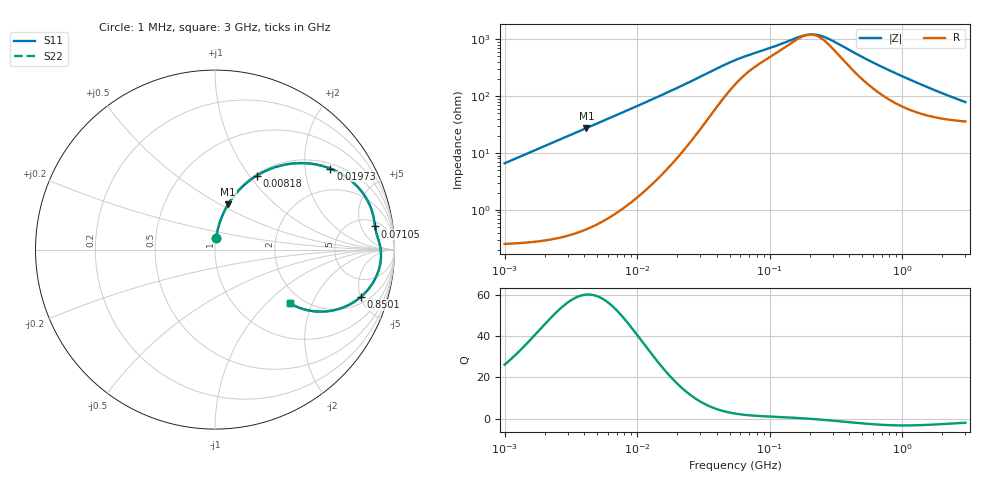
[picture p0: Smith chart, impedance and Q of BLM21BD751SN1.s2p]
! BLM21BD751SN1
# Hz S RI R 50
!Freq.(Hz) S11(Real) S11(Imag) S21(Real) S21(Imag) S12(Real) S12(Imag) S22(Real) S22(Imag)
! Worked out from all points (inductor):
!   401 points, 1 MHz to 3 GHz, reference 50 ohm
!   read as one part in series: L = 1.05 uH near 1.041 MHz
!   highest Q = 60 at 4.142 MHz (marker M1), where L = 1.05 uH
!   self-resonance near 198.1 MHz
!   S11 on the Smith chart (normalised r, x): 1 MHz: 1.01, +0.13; 8.18 MHz: 1.02, +1.09; 19.73 MHz: 1.16, +2.73; 71.05 MHz: 7, +9; 850.1 MHz: 2.59, -5.06; 3 GHz: 1.72, -1.40
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1000000  0.0068 0.0653  0.9932 -0.0653  0.9932 -0.0653  0.0068 0.0653
2014875  0.0201 0.1297  0.9799 -0.1297  0.9799 -0.1297  0.0201 0.1297
3823119  0.0633 0.2353  0.9367 -0.2353  0.9367 -0.2353  0.0633 0.2353
4141799  0.0732 0.2522  0.9268 -0.2522  0.9268 -0.2522  0.0732 0.2522
5938264  0.1382 0.3363  0.8618 -0.3363  0.8618 -0.3363  0.1382 0.3363
8179831  0.2329 0.4123  0.7671 -0.4123  0.7671 -0.4123  0.2329 0.4123
1.126754e7  0.3666 0.4682  0.6334 -0.4682  0.6334 -0.4682  0.3666 0.4682
1.461624e7  0.4954 0.4816  0.5046 -0.4816  0.5046 -0.4816  0.4954 0.4816
1.973457e7  0.6434 0.4512  0.3566 -0.4512  0.3566 -0.4512  0.6434 0.4512
2.559965e7  0.7503 0.3904  0.2497 -0.3904  0.2497 -0.3904  0.7503 0.3904
3.254976e7  0.8205 0.3192  0.1795 -0.3192  0.1795 -0.3192  0.8205 0.3192
5.477226e7  0.8843 0.1766  0.1157 -0.1766  0.1157 -0.1766  0.8843 0.1766
7.105049e7  0.8917 0.1292  0.1083 -0.1292  0.1083 -0.1292  0.8917 0.1292
1.680187e8  0.9193 0.0224  0.0807 -0.0224  0.0807 -0.0224  0.9193 0.0224
2.094008e8  0.9239 -0.00786  0.0761 0.00786  0.0761 0.00786  0.9239 -0.00786
2.361213e8  0.9249 -0.0255  0.0751 0.0255  0.0751 0.0255  0.9249 -0.0255
2.716345e8  0.9245 -0.047  0.0755 0.047  0.0755 0.047  0.9245 -0.047
4.951867e8  0.8966 -0.1537  0.1034 0.1537  0.1034 0.1537  0.8966 -0.1537
8.005644e8  0.8262 -0.2511  0.1738 0.2511  0.1738 0.2511  0.8262 -0.2511
8.501091e8  0.8132 -0.2629  0.1868 0.2629  0.1868 0.2629  0.8132 -0.2629
1.613037e9  0.6192 -0.3443  0.3808 0.3443  0.3808 0.3443  0.6192 -0.3443
3e9  0.4175 -0.2996  0.5825 0.2996  0.5825 0.2996  0.4175 -0.2996
